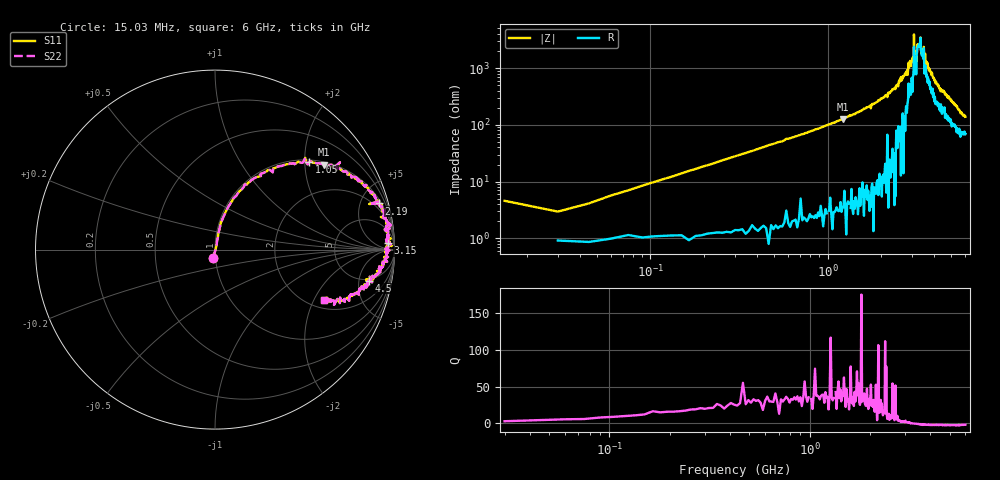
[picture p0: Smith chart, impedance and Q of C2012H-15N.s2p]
!	Network	Analyzer	HP8753E.07.74:	Oct	30	2002	Serial	No.	JP38451487
!	Hewlett-Packard
!	28	Aug	2009	9:49:57
!	Frequency	S11	S21	S12	S22
#	HZ	S	RI	R	50
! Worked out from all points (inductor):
!   400 points, 15.03 MHz to 6 GHz, reference 50 ohm
!   read as one part in series: L = 14.7 nH near 45.03 MHz
!   highest Q = 38.8 at 1.215 GHz (marker M1), where L = 16.4 nH
!   self-resonance near 3.309 GHz
!   S11 on the Smith chart (normalised r, x): 15.03 MHz: 0.98, -0.09; 1.05 GHz: 1.05, +2.10; 2.19 GHz: 1.36, +6.98; 3.15 GHz: 27, +29; 4.5 GHz: 4.67, -6.91; 6 GHz: 2.39, -2.41
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1.502992e7  -0.0092 -0.0455  1.01 0.0455  1.01 0.0455  -0.0092 -0.0455
3.002985e7  0.00976 0.0277  0.99 -0.0277  0.99 -0.0277  0.00976 0.0277
1.200294e8  0.0229 0.108  0.977 -0.108  0.977 -0.108  0.0229 0.108
3.300284e8  0.0967 0.273  0.903 -0.273  0.903 -0.273  0.0967 0.273
1.020025e9  0.509 0.485  0.491 -0.485  0.491 -0.485  0.509 0.485
1.050025e9  0.525 0.487  0.475 -0.487  0.475 -0.487  0.525 0.487
1.215024e9  0.609 0.474  0.391 -0.474  0.391 -0.474  0.609 0.474
2.01002e9  0.885 0.304  0.115 -0.304  0.115 -0.304  0.885 0.304
2.190019e9  0.913 0.257  0.0872 -0.257  0.0872 -0.257  0.913 0.257
3.015015e9  0.98 0.0615  0.02 -0.0615  0.02 -0.0615  0.98 0.0615
3.060015e9  0.966 0.0481  0.0338 -0.0481  0.0338 -0.0481  0.966 0.0481
3.075015e9  0.984 0.0197  0.0157 -0.0197  0.0157 -0.0197  0.984 0.0197
3.105014e9  0.96 0.054  0.0397 -0.054  0.0397 -0.054  0.96 0.054
3.150014e9  0.965 0.0354  0.0353 -0.0354  0.0353 -0.0354  0.965 0.0354
3.345013e9  0.972 -0.00449  0.0277 0.00449  0.0277 0.00449  0.972 -0.00449
3.405013e9  0.947 -0.0139  0.053 0.0139  0.053 0.0139  0.947 -0.0139
3.495013e9  0.962 -0.0131  0.0385 0.0131  0.0385 0.0131  0.962 -0.0131
3.525012e9  0.946 -0.0558  0.0544 0.0558  0.0544 0.0558  0.946 -0.0558
4.00501e9  0.921 -0.126  0.0792 0.126  0.0792 0.126  0.921 -0.126
4.500008e9  0.858 -0.173  0.142 0.173  0.142 0.173  0.858 -0.173
5.010005e9  0.799 -0.237  0.201 0.237  0.201 0.237  0.799 -0.237
6e9  0.608 -0.279  0.392 0.279  0.392 0.279  0.608 -0.279
